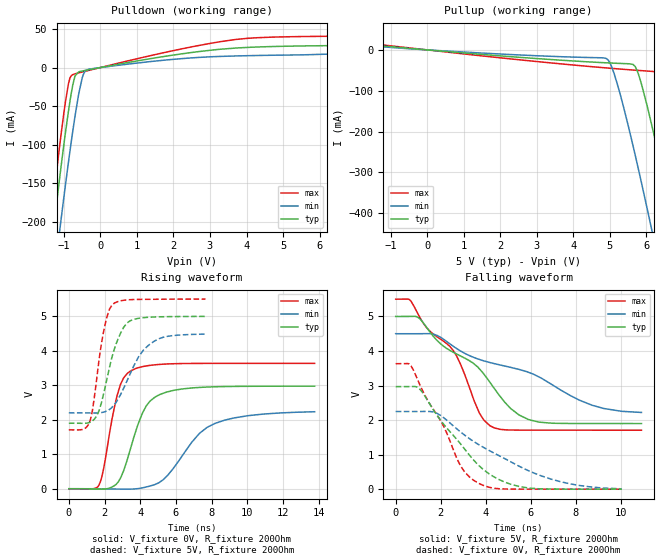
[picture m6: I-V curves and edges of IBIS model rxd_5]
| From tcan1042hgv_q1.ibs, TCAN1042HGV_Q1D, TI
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|   rxd_5 Model
[Model]   rxd_5
Model_type   Output
Polarity   Non-Inverting
Vmeas = 2.5
Vref = 0
Cref = 2pF
Rref = 250
|   typ   min   max
|   (nom PVT)   (fast PVT)   (slow PVT)
C_comp   2.386e-12   2.168e-12   2.894e-12
| Where nom  PVT is Nominal Process, 5V, 27C
|   Fast PVT is Strong Process,  5.5V, -55C
|   Slow PVT is Weak Process,   4.5V, 150C
[Voltage Range]   5   4.5   5.5
|Junction Temperature
[Temperature Range]   27   150   -55
[Pullup Reference]   5   4.5   5.5
[Pulldown Reference]   0   0   0
[Power Clamp Reference]   5   4.5   5.5
[GND Clamp Reference]   0   0   0
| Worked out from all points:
|   slope of the pulldown table from 0 to 0.75 V, typ, clamps not added: 115 ohm
|   slope of the pullup table from 0 to 0.75 V, typ, clamps not added: 132 ohm
|   falling waveform, V_fixture 5V, R_fixture 200Ohm: 20-80 % time 3.11ns typ, 5.09ns min, 2.25ns max; typ from 5 V to 1.9 V
|   rising waveform, V_fixture 0V, R_fixture 200Ohm: 20-80 % time 1.2ns typ, 2.14ns min, 823ps max; typ from 0 V to 2.97 V
|   rising waveform, V_fixture 5V, R_fixture 200Ohm: 20-80 % time 946ps typ, 1.37ns min, 646ps max; typ from 1.9 V to 5 V
|   falling waveform, V_fixture 0V, R_fixture 200Ohm: 20-80 % time 2.25ns typ, 3.56ns min, 1.68ns max; typ from 2.97 V to 0.001 V
[Pulldown]
|   Voltage   I(typ)   I(min)   I(max)
-5V       -1.938A    -1.963A    -1.932A
-1.377V   -248.8mA   -316mA     -209.1mA
-1.13V    -148.8mA   -217.5mA   -107.2mA
-1.073V   -127mA     -195.6mA   -85.47mA
-875mV    -56.91mA   -122.9mA   -21.26mA
-702.5mV  -12.29mA   -65.58mA   -8.197mA
-500mV    -4.424mA   -13.85mA   -5.745mA
-324.5mV  -2.846mA   -2.215mA   -3.716mA
3.728V    25.37mA    15.1mA     36.53mA
6.803V    28.7mA     18.18mA    40.78mA
8.045V    29.33mA    26.87mA    41.11mA
10V       47.12mA    41.2mA     50.1mA
[Pullup]
|   Voltage   I(typ)   I(min)   I(max)
-5V       40.48mA    32.39mA    49.71mA
4.886V    -31.59mA   -20.71mA   -44.08mA
5.115V    -32.54mA   -58.15mA   -45.76mA
5.63V     -35.43mA   -233.7mA   -49.34mA
5.818V    -69.8mA    -307.1mA   -50.55mA
6.025V    -138.9mA   -390.8mA   -51.84mA
6.191V    -202mA     -459.7mA   -52.94mA
6.357V    -268.5mA   -529.6mA   -63.55mA
6.72V     -421.4mA   -685.5mA   -189.1mA
7.105V    -590.7mA   -855.6mA   -352.4mA
7.405V    -725.6mA   -991.5mA   -486.5mA
10V       -1.941A    -2.202A    -1.705A
[Ramp]
R_load = 200
|   typ   min   max
dV/dt_r   1.78423/1.19645e-09   1.35379/2.20652e-09   2.1811/8.22747e-10
dV/dt_f   1.86055/3.10845e-09   1.38029/5.12898e-09   2.27576/2.25078e-09
[Falling Waveform]
V_fixture = 5V
V_fixture_min = 4.5V
V_fixture_max = 5.5V
R_fixture = 200Ohm
|   Time   V(typ)   V(min)   V(max)
0s        5V         4.5V       5.5V
597.3ps   5.001V     4.5V       5.494V
1.021ns   4.959V     4.5V       5.033V
2.562ns   3.961V     4.136V     4.01V
3.717ns   3.485V     3.756V     2.204V
4.187ns   3.093V     3.666V     1.837V
5.102ns   2.338V     3.527V     1.713V
5.898ns   2.016V     3.384V     1.709V
8.726ns   1.9V       2.429V     1.708V
10.92ns   1.9V       2.221V     1.707V
[Rising Waveform]
V_fixture = 0V
V_fixture_min = 0V
V_fixture_max = 0V
R_fixture = 200Ohm
|   Time   V(typ)   V(min)   V(max)
0s        83.56pV    37.66nV    52.85pV
1.696ns   -11.4mV    -764.2uV   113.6mV
1.945ns   -10.34mV   -2.302mV   569mV
2.708ns   162.5mV    -8.668mV   2.71V
3.474ns   1.198V     -10.36mV   3.419V
4.337ns   2.405V     51.96mV    3.561V
5.472ns   2.803V     358.2mV    3.617V
7.316ns   2.937V     1.606V     3.634V
8.161ns   2.956V     1.89V      3.635V
13.76ns   2.973V     2.232V     3.635V
[Rising Waveform]
V_fixture = 5V
V_fixture_min = 4.5V
V_fixture_max = 5.5V
R_fixture = 200Ohm
|   Time   V(typ)   V(min)   V(max)
0s        1.899V     2.2V       1.707V
871.2ps   1.897V     2.199V     1.742V
1.21ns    1.933V     2.197V     1.999V
1.551ns   2.101V     2.196V     3.146V
1.945ns   2.746V     2.222V     4.548V
2.407ns   3.799V     2.355V     5.319V
3.243ns   4.798V     3.11V      5.475V
4.469ns   4.972V     4.164V     5.492V
5.531ns   4.989V     4.42V      5.496V
7.654ns   4.997V     4.484V     5.5V
[Falling Waveform]
V_fixture = 0V
V_fixture_min = 0V
V_fixture_max = 0V
R_fixture = 200Ohm
|   Time   V(typ)   V(min)   V(max)
0s        2.969V     2.248V     3.633V
597.3ps   2.97V      2.248V     3.626V
1.021ns   2.925V     2.249V     3.099V
1.854ns   2.122V     2.19V      2.131V
2.884ns   1.309V     1.655V     668.9mV
3.717ns   672.3mV    1.28V      159mV
4.836ns   207.1mV    887.3mV    5.685mV
5.898ns   34.39mV    535.8mV    1.224mV
7.747ns   1.562mV    154.6mV    636.8uV
10.04ns   719.3uV    10.71mV    385.9uV
